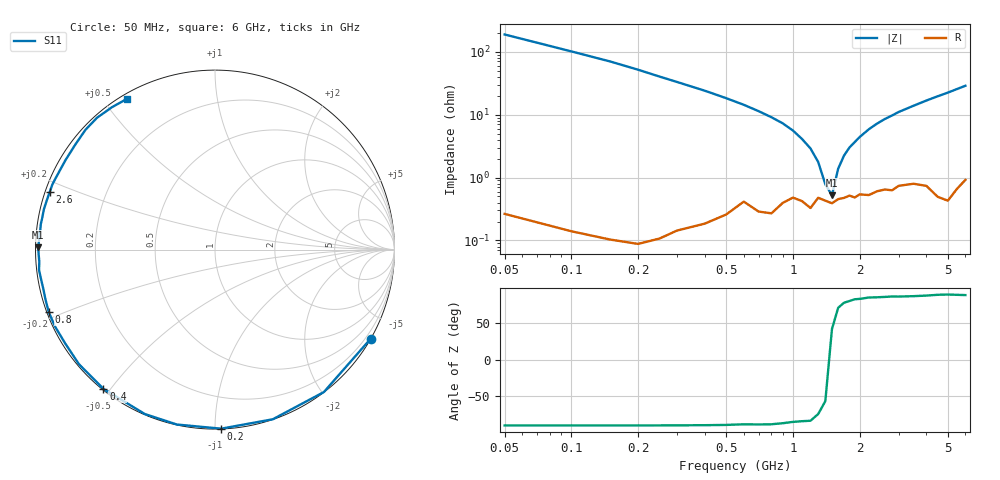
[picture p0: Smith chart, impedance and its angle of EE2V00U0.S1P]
! Infineon Technologies  Discrete & RF Semiconductors
! BBY55-02W
! Si Tuning Diode in SCD-80
! VR = 2 V
! S-Parameters:  June  2000
# GHz  S  MA  R  50
!  f  S11
! GHz  MAG  ANG
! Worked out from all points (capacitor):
!   34 points, 50 MHz to 6 GHz, reference 50 ohm
!   read as one part to ground: C = 15.7 pF near 50 MHz
!   lowest |Z| = 524 mohm at 1.5 GHz (marker M1)
!   series resonance near 1.465 GHz, so ESL is about 750 pH
!   S11 on the Smith chart (normalised r, x): 50 MHz: 0.01, -3.76; 200 MHz: 0.00, -1.04; 400 MHz: 0.00, -0.48; 800 MHz: 0.01, -0.18; 2.6 GHz: 0.01, +0.17; 6 GHz: 0.02, +0.57
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0.05  0.9993 -29.8
0.1  0.9989 -52.6
0.15  0.9986 -71.2
0.2  0.9983 -88.0
0.25  0.9974 -102.3
0.3  0.996 -113.1
0.4  0.994 -128.7
0.5  0.9909 -139.9
0.6  0.9848 -148.0
0.7  0.9891 -154.4
0.8  0.9896 -159.4
1  0.9812 -167.3
1.1  0.9834 -170.7
1.2  0.987 -173.4
1.3  0.9811 -176.1
1.5  0.9845 179.2
1.6  0.982 177.0
1.8  0.9796 173.2
2.2  0.9794 166.7
2.4  0.9765 163.6
2.6  0.9752 160.7
3  0.9722 155.2
3.5  0.9708 149.1
4  0.9738 143.0
4.5  0.983 137.2
5  0.9858 131.8
5.5  0.9792 125.9
6  0.9728 120.2
